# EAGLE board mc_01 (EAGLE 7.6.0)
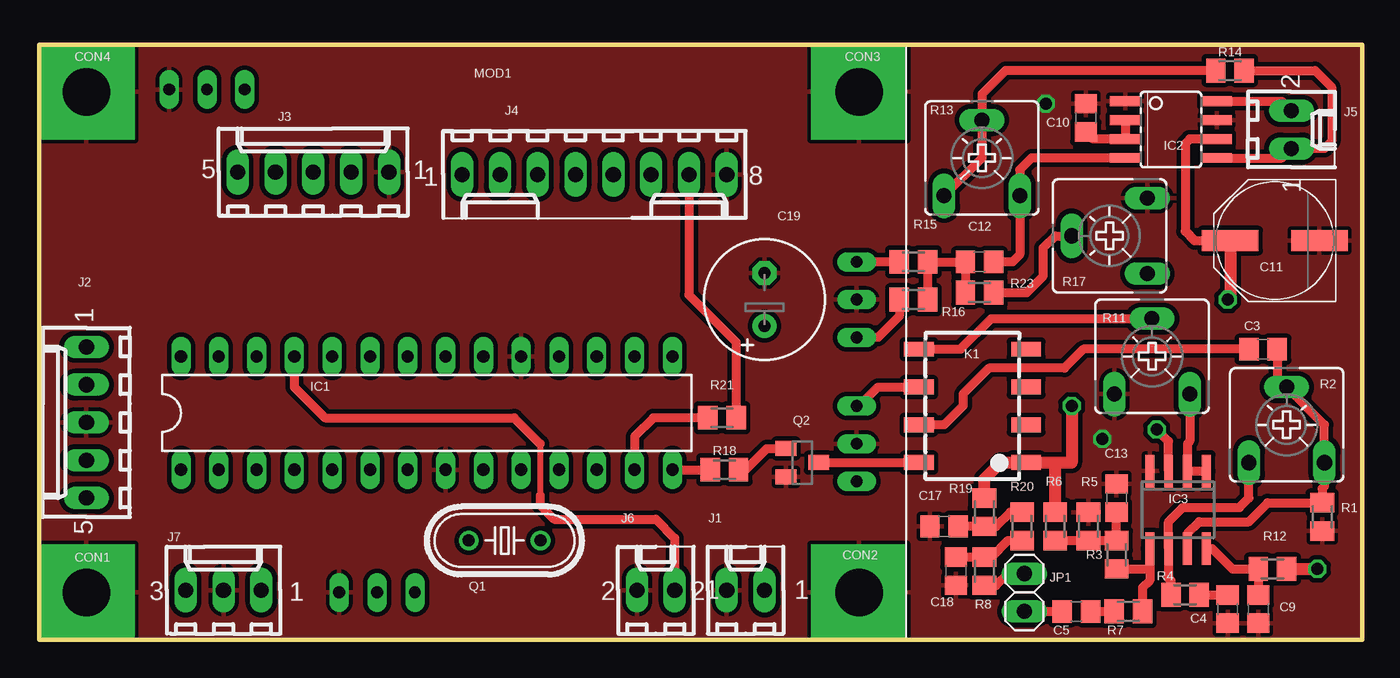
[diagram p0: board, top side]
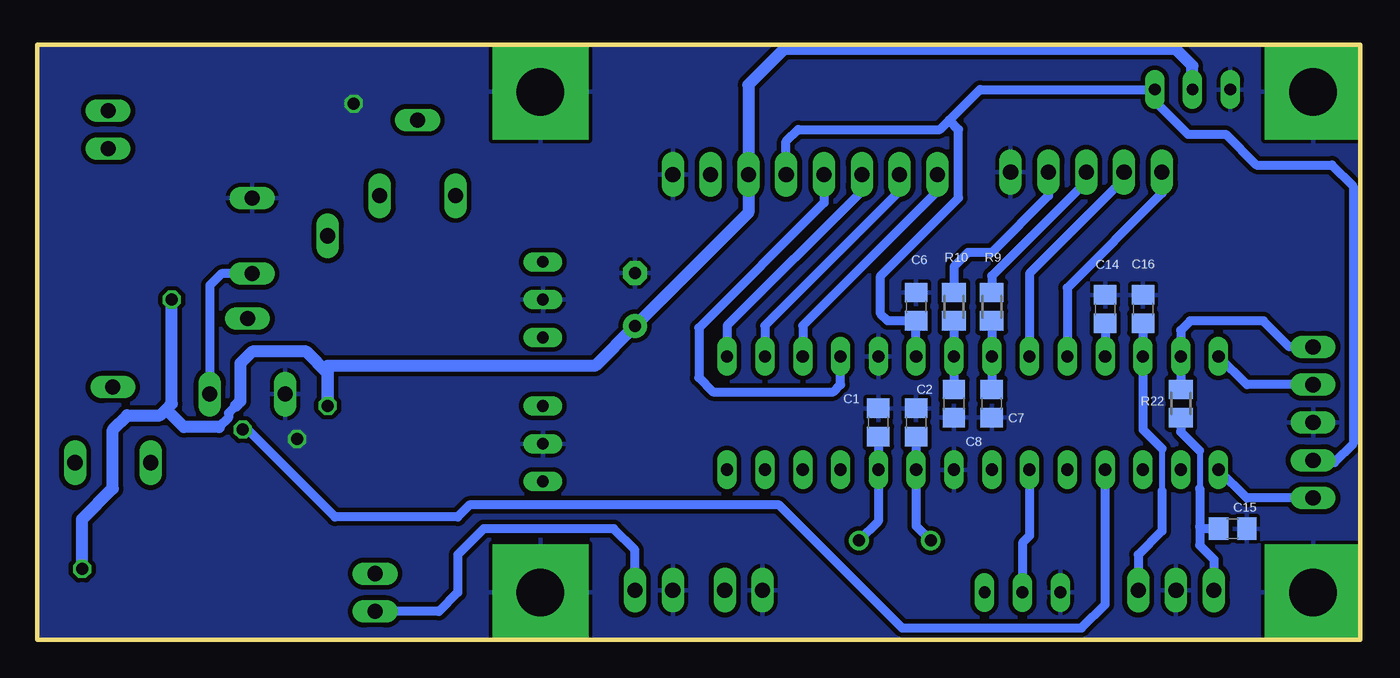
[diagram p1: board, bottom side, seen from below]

Size 88.9 x 40.01 mm. Coordinates in mm from the lower left corner, seen from the top.
Outline: 0,0 88.9,0 88.9,40.01 0,40.01 0,0
Copper layers (1*16): Top 0.035mm / dielectric 1.5mm / Bottom 0.035mm
Design rules "default *": minimum track width 10mil, minimum drill 24mil, track to track 8mil, track to pad 8mil, pad to pad 8mil, via to via 8mil, smd to smd 8mil, copper to edge 0mil, drill to drill 8mil, minimum pad ring 10mil, minimum via ring 8mil, stop-mask expansion 4mil, vias tented up to drill 0mil, thermal gap 10mil

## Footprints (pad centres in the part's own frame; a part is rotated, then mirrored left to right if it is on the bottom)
C0805 = smd 1.3 x 1.5: 1 -0.95,0; 2 0.95,0
PANASONIC_E = smd 3.8 x 1.4: + 3,0; - -3,0
E3,5-8 = drill 0.813 pad 1.6: + -1.778,0 | drill 0.813 pad 1.6 octagon: - 1.778,0
HOLE3 = drill 3.2 pad 6.452 square: 1 0,0
DIL28-3 = drill 0.813 long: 1 -16.51,-3.81; 2 -13.97,-3.81; 3 -11.43,-3.81; 4 -8.89,-3.81; 5 -6.35,-3.81; 6 -3.81,-3.81; 7 -1.27,-3.81; 8 1.27,-3.81; 9 3.81,-3.81; 10 6.35,-3.81; 11 8.89,-3.81; 12 11.43,-3.81; 13 13.97,-3.81; 14 16.51,-3.81; 15 16.51,3.81; 16 13.97,3.81; 17 11.43,3.81; 18 8.89,3.81; 19 6.35,3.81; 20 3.81,3.81; 21 1.27,3.81; 22 -1.27,3.81; 23 -3.81,3.81; 24 -6.35,3.81; 25 -8.89,3.81; 26 -11.43,3.81; 27 -13.97,3.81; 28 -16.51,3.81
SOIC08 = smd 0.66 x 2.032: 1 -1.905,-3.073; 2 -0.635,-3.073; 3 0.635,-3.073; 4 1.905,-3.073; 5 1.905,3.073; 6 0.635,3.073; 7 -0.635,3.073; 8 -1.905,3.073
SO08 = smd 0.6 x 2.2: 1 -1.905,-2.6; 2 -0.635,-2.6; 3 0.635,-2.6; 4 1.905,-2.6; 5 1.905,2.6; 6 0.635,2.6; 7 -0.635,2.6; 8 -1.905,2.6
6410-02 = drill 1.016 long: 1 1.27,0; 2 -1.27,0
6410-05 = drill 1.016 long: 1 5.08,0; 2 2.54,0; 3 0,0; 4 -2.54,0; 5 -5.08,0
6410-08 = drill 1.016 long: 1 8.89,0; 2 6.35,0; 3 3.81,0; 4 1.27,0; 5 -1.27,0; 6 -3.81,0; 7 -6.35,0; 8 -8.89,0
6410-03 = drill 1.016 long: 1 2.54,0; 2 0,0; 3 -2.54,0
1X02 = drill 1.016 long: 1 -1.27,0; 2 1.27,0
G6K-2F = smd 1 x 2: 1 -3.81,-3.6; 2 -1.27,-3.6; 3 1.27,-3.6; 4 3.81,-3.6; 5 3.81,3.6; 6 1.27,3.6; 7 -1.27,3.6; 8 -3.81,3.6
USB_QO100 = drill 0.8 long: 1 8.731,36.989; 2 11.271,36.989; 3 20.161,3.175; 4 22.701,3.175; 5 25.241,3.175; 6 54.928,25.4; 7 54.928,22.86; 8 54.928,20.32; 9 54.928,15.716; 10 54.928,13.176; 11 54.928,10.636; 12 13.811,36.989
HC49U-V = drill 0.813: 1 -2.413,0; 2 2.413,0
SOT23 = smd 1 x 1.4: 1 -0.95,-1.1; 2 0.95,-1.1; 3 0,1.1
M0805 = smd 1.3 x 1.6: 1 -0.95,0; 2 0.95,0
CA6V = drill 1.016 long: A -2.54,-2.54; E 2.54,-2.54; S 0,2.54

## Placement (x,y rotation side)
C1  27p  [C0805]  32.38,14.61 270 bottom
C2  27p  [C0805]  29.84,14.61 270 bottom
C3  1u  [C0805]  82.23,19.53 0 top
C4  10u  [C0805]  79.85,2.06 270 top
C5  1u  [C0805]  69.69,1.91 180 top
C6  100n  [C0805]  29.84,22.38 90 bottom
C7  100n  [C0805]  24.77,15.88 90 bottom
C8  100n  [C0805]  27.3,15.88 90 bottom
C9  10u  [C0805]  81.92,2.06 270 top
C10  1u  [C0805]  70.33,35.08 90 top
C11  47u  [PANASONIC_E]  83.03,26.83 180 top
C12  100n  [C0805]  63.18,25.4 180 top
C13  10u  [C0805]  72.39,9.53 270 top
C14  1n  [C0805]  17.14,22.23 270 bottom
C15  1n  [C0805]  8.57,7.46 0 bottom
C16  1n  [C0805]  14.61,22.23 270 bottom
C17  10u  [C0805]  60.8,7.62 0 top
C18  10u  [C0805]  61.59,4.6 90 top
C19  470u  [E3,5-8]  48.74,22.86 90 top
CON1  [HOLE3]  3.17,3.17 0 top
CON2  [HOLE3]  55.09,3.17 0 top
CON3  [HOLE3]  55.09,36.83 0 top
CON4  [HOLE3]  3.17,36.83 0 top
IC1  PIC18F26K22  [DIL28-3]  26.04,15.24 0 top
IC2  TPA4861  [SOIC08]  76.04,34.29 270 top
IC3  AD823  [SO08]  76.52,8.73 180 top
J1  Mike  [6410-02]  47.47,3.33 0 top
J2  Programmer  [6410-05]  3.17,14.61 90 top
J3  Drehgeber  [6410-05]  18.41,31.43 0 top
J4  LCD  [6410-08]  37.31,31.27 180 top
J5  LP  [6410-02]  84.14,34.29 270 top
J6  PTT  [6410-02]  41.43,3.33 0 top
J7  Keyer  [6410-03]  12.38,3.33 0 top
JP1  Speisung  [1X02]  66.2,3.17 270 top
K1  G6K-2F  [G6K-2F]  62.71,15.72 90 top
MOD1  USB-Modul  [USB_QO100]  0,0 0 top
Q1  16 MHz  [HC49U-V]  31.27,6.67 180 top
Q2  BSS123  [SOT23]  51.28,11.91 270 top
R1  10k  [M0805]  86.2,8.26 270 top
R2  22k  [CA6V]  83.82,14.45 0 top
R3  4,7k  [M0805]  72.39,5.71 90 top
R4  220  [M0805]  76.99,3.02 180 top
R5  4,7k  [M0805]  70.48,7.62 270 top
R6  4,7k  [M0805]  68.26,7.62 90 top
R7  1k  [M0805]  73.18,1.91 0 top
R8  2,2k  [M0805]  63.5,4.6 270 top
R9  100  [M0805]  24.77,22.38 90 bottom
R10  100  [M0805]  27.3,22.38 90 bottom
R11  50k  [CA6V]  74.77,19.05 0 top
R12  47  [M0805]  82.87,4.76 0 top
R13  100k  [CA6V]  63.34,32.38 0 top
R14  27k  [M0805]  80.01,38.26 0 top
R15  10k  [M0805]  58.74,25.4 0 top
R16  10k  [M0805]  58.74,22.86 0 top
R17  220k  [CA6V]  71.91,27.15 90 top
R18  4,7k  [M0805]  46.04,11.43 180 top
R19  1k  [M0805]  63.5,8.57 270 top
R20  1k  [M0805]  66.04,7.62 270 top
R21  180  [M0805]  45.88,14.92 0 top
R22  470  [M0805]  12.06,15.88 270 bottom
R23  10k  [M0805]  63.18,23.34 180 top

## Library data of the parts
C1-C19 R1 R3-R10 R12 R14-R16 R18-R23 = rcl
CON1-CON4 IC2 MOD1 = lindenau
IC1 = microchip; MF: MICROCHIP; MPN: PIC18F2550-I/SP; OC_FARNELL: 1523822; OC_NEWARK: 80K6054
IC3 = linear
J1-J7 = con-molex; OC_FARNELL: unknown; OC_NEWARK: unknown
JP1 = pinhead
K1 = relay; MF: OMRON COMPONENTS USA; MPN: G6K-2F DC24; OC_FARNELL: 1690427; OC_NEWARK: 36K7467
Q1 = crystal; OC_FARNELL: 1666969; OC_NEWARK: unknown
Q2 = transistor-small-signal
R2 R11 R13 R17 = pot

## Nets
5V: C11.+ C19.+ IC2.6 J4.6 K1.1 MOD1.2 R6.2 R12.2 R19.1
GND: C1.1 C2.1 C4.2 C6.2 C7.1 C8.1 C9.2 C10.2 C11.- C13.1 C14.1 C15.2 C16.1 C17.1 C18.1 C19.- CON1.1 CON2.1 CON3.1 CON4.1 IC1.8 IC1.19 IC2.1 IC2.7 IC3.4 J1.2 J2.3 J3.1 J4.8 J6.2 J7.2 MOD1.1 MOD1.3 MOD1.7 MOD1.10 Q2.2 R1.2 R5.1 R11.A R17.E
MCLR: IC1.1 J2.5
MIKE: C5.2 J1.1 JP1.2
N$1: J3.3 R9.2
N$2: IC3.1 IC3.2 R11.E R17.A
N$3: K1.6 MOD1.9
N$4: J3.2 R10.2
N$5: C10.1 IC2.2 IC2.3
N$6: R13.A R13.S R14.1
N$7: IC2.5 J5.1 R14.2
N$8: C9.1 IC3.8 R12.1
N$9: K1.5 R11.S
N$10: C2.2 IC1.9 Q1.2
N$11: C12.1 IC2.4 R13.E
N$12: C1.2 IC1.10 Q1.1
N$13: MOD1.6 R15.1
N$14: MOD1.8 R16.1
N$15: C12.2 R15.2 R16.2 R23.2
N$16: IC2.8 J5.2
N$17: K1.8 Q2.3
N$18: Q2.1 R18.1
N$19: C3.2 IC3.7 R1.1 R2.E R2.S
N$20: C18.2 R8.1 R20.2
N$21: C17.2 R19.2 R20.1
N$22: JP1.1 R8.2
N$23: J4.7 R21.2
N$24: R17.S R23.1
N$30: C5.1 R7.1
N$62: IC3.6 R2.A R4.2
N$63: C4.1 R4.1
N$64: C13.2 R3.2 R5.2 R6.1
N$65: IC3.5 R3.1 R7.2
N$76: C3.1 K1.7
RA0: IC1.2
RA1: IC1.3
RA2: IC1.4 IC3.3
RA3: IC1.5
RA4: IC1.6 MOD1.4
RA5: IC1.7
RB0: C8.2 IC1.21 R10.1
RB1: C7.2 IC1.22 R9.1
RB2: IC1.23 J3.4
RB3: IC1.24 J3.5
RB4: C14.2 IC1.25 J6.1
RB5: C16.2 IC1.26 J7.1
RB6: IC1.27 J2.1 R22.1
RB6_1: C15.1 J7.3 R22.2
RB7: IC1.28 J2.2
RC0: IC1.11
RC1: IC1.12
RC2: IC1.13 R21.1
RC3: IC1.14 R18.2
RC4: IC1.15 J4.3
RC5: IC1.16 J4.2
RC6: IC1.17 J4.1
RC7: IC1.18 J4.4
VDD: C6.1 IC1.20 J2.4 J4.5 MOD1.12

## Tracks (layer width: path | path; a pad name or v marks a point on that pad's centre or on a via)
5V  (via drill 0.8)
  Top 0.61: 66.2,11.8 K1.1 | IC2.6 77.31,33.66 76.99,33.34 76.99,27.46 77.63,26.83 C11.+
  Top 0.813: 68.1,11.91 K1.1 64.61,11.91 63.5,10.79 R19.1 | 68.1,11.91 69.37,11.91 v69.37,15.72 | R12.2 v85.88,4.76 | C11.+ 80.03,23.04 v79.85,22.86 | R6.2 68.26,11.75 68.1,11.91
  Bottom 0.61: 75.56,15.72 76.04,15.24 76.04,14.92 76.68,14.29
  Bottom 0.813: MOD1.2 11.27,38.58 12.38,39.69 38.73,39.69 41.12,37.31 J4.6 41.12,28.7 C19.+ 48.77,21.08 51.44,18.41 69.37,18.41 v69.37,15.72 69.37,17.94 70.8,19.37 74.45,19.37 75.25,18.57 75.25,16.03 75.56,15.72 | v85.88,4.76 85.88,8.1 83.82,10.16 83.82,14.13 82.87,15.08 80.64,15.08 80.25,15.48 | 80.25,15.48 79.85,15.88 v79.85,22.86 | 76.68,14.29 79.06,14.29 80.25,15.48
GND  (via drill 0.8)
  other vias: 71.44,13.49 67.63,36.04
  pour Bottom (isolate 0.305): 0,0 0,40.01 88.9,40.01 88.9,0
  pour Top (isolate 0.305): 0,0 0,40.01 88.9,40.01 88.9,0
MCLR
  Bottom 0.61: J2.5 7.62,9.53 IC1.1
MIKE
  Top 0.61: JP1.2 C5.2
  Bottom 0.61: J1.1 48.74,6.03 50.16,7.46 58.9,7.46 60.64,5.71 60.64,3.17 61.91,1.91 JP1.2
N$1
  Bottom 0.61: J3.3 18.41,30.8 24.77,24.45 R9.2
N$2
  Top 0.61: IC3.1 IC3.2 77.15,13.18 77.31,13.34 R11.E
  Bottom 0.61: R17.A 76.52,24.61 77.31,23.81 R11.E
N$3
  Top 0.61: MOD1.9 55.09,15.72 56.36,16.99 K1.6
N$4
  Bottom 0.61: J3.2 20.95,29.84 24.77,26.04 26.35,26.04 27.3,25.08 R10.2
N$5
  Top 0.61: C10.1 70.81,33.66 IC2.3 IC2.2
N$6
  Top 0.61: R13.A 63.34,32.38 R13.S 63.34,36.67 64.93,38.26 R14.1
N$7
  Top 0.61: IC2.5 83.5,32.38 J5.1 86.36,33.02 86.84,33.5 86.84,37.15 85.72,38.26 R14.2
N$8
  Top 0.61: 81.92,2.86 C9.1 R12.1 80.17,4.76 78.8,6.13 IC3.8
N$9
  Top 0.61: K1.5 61.91,19.53 63.98,21.59 R11.S 74.93,21.75
N$10
  Bottom 0.61: Q1.2 29.84,7.65 IC1.9 C2.2
N$11
  Top 0.61: C12.1 65.41,25.4 65.88,25.88 R13.E 65.88,31.59 66.67,32.38 IC2.4
N$12
  Bottom 0.61: Q1.1 32.38,7.97 IC1.10 C1.2
N$13
  Top 0.61: R15.1 MOD1.6
N$14
  Top 0.61: R16.1 57.79,21.75 56.36,20.32 MOD1.8
N$15
  Top 0.61: R16.2 R15.2 C12.2 R23.2
N$16
  Top 0.61: IC2.8 83.5,36.2 J5.2
N$17
  Top 0.61: Q2.3 K1.8
N$18
  Top 0.61: R18.1 47.47,11.43 48.9,12.86 Q2.1
N$19
  Top 0.61: IC3.7 77.15,7.14 77.95,7.94 81.28,7.94 82.55,9.21 R1.1 86.2,10.16 86.36,10.32 R2.E 86.36,14.45 R2.S 83.18,17.62 C3.2
N$20
  Top 0.61: C18.2 R8.1 63.97,5.55 65.09,6.67 R20.2
N$21
  Top 0.61: R20.1 65.24,8.57 64.29,7.62 R19.2 C17.2
N$22
  Top 0.61: R8.2 64.3,3.65 65.09,4.45 JP1.1
N$23
  Top 0.61: J4.7 43.66,23.18 46.83,20 R21.2
N$24
  Top 0.61: R23.1 66.36,23.34 67.47,24.45 67.47,26.35 68.26,27.15 R17.S
N$30
  Top 0.61: C5.1 R7.1
N$62
  Top 0.61: R2.A 81.28,9.53 80.64,8.89 76.83,8.89 75.88,7.94 IC3.6 75.88,4.13 76.04,3.97 R4.2
N$63
  Top 0.61: R4.1 C4.1
N$64
  Top 0.61: R6.1 R5.2 R3.2 C13.2
N$65
  Top 0.61: IC3.5 74.61,4.6 | 74.61,4.6 74.61,3.97 74.14,3.49 R7.2 | R3.1 74.45,4.76 74.61,4.6
N$76
  Top 0.61: C3.1 70.17,19.53 68.9,18.26 63.82,18.26 62.07,16.51 62.07,15.72 60.8,14.45 K1.7
RA2  (via drill 0.8)
  Top 0.61: IC3.3 75.88,13.34 v75.09,14.13
  Bottom 0.61: v75.09,14.13 74.77,14.13 68.9,8.26 60.64,8.26 59.85,9.05 39.05,9.05 30.8,0.79 18.73,0.79 17.14,2.38 IC1.4
RA4
  Bottom 0.61: IC1.6 22.23,6.99 22.7,6.51 MOD1.4
RB0
  Bottom 0.61: R10.1 IC1.21 C8.2
RB1
  Bottom 0.61: R9.1 IC1.22 C7.2
RB2
  Bottom 0.61: J3.4 15.88,30.96 22.23,24.61 IC1.23
RB3
  Bottom 0.61: J3.5 13.34,30 19.68,23.65 IC1.24
RB4
  Top 0.406: 33.66,13.18 33.66,9.68
  Top 0.61: IC1.25 17.14,16.99 19.21,14.92 31.91,14.92 33.66,13.18 | 33.66,9.68 33.66,9.05 34.61,8.1 41.43,8.1 42.7,6.83 J6.1
  Bottom 0.61: C14.2 IC1.25
RB5
  Bottom 0.406: 13.34,12.86 13.34,10
  Bottom 0.61: C16.2 IC1.26 14.61,14.13 13.34,12.86 | 13.34,10 13.34,7.3 14.92,5.71 J7.1
RB6
  Bottom 0.61: J2.1 4.76,19.68 6.51,21.43 11.43,21.43 12.06,20.8 IC1.27 R22.1
RB6_1
  Bottom 0.406: 10.79,12.7 10.79,10.16
  Bottom 0.61: R22.2 12.06,13.97 10.79,12.7 | 10.79,10.16 10.79,7.62 | 10.79,7.62 10.79,6.35 9.84,5.4 J7.3 | C15.1 10.64,7.46 10.79,7.62
RB7
  Bottom 0.61: J2.2 7.62,17.14 IC1.28
RC2
  Top 0.61: R21.1 41.27,14.92 40.01,13.65 IC1.13
RC3
  Top 0.61: IC1.14 R18.2
RC4
  Bottom 0.61: J4.3 33.5,30.16 42.55,21.11 IC1.15
RC5
  Bottom 0.61: J4.2 30.96,30.16 40.01,21.11 IC1.16
RC6
  Bottom 0.61: J4.1 28.42,30.16 37.47,21.11 IC1.17
RC7
  Bottom 0.61: J4.4 36.04,29.37 44.45,20.95 44.45,17.62 43.5,16.67 35.4,16.67 34.92,17.14 IC1.18
VDD
  Bottom 0.61: J4.5 38.58,33.5 37.78,34.29 28.26,34.29 27.62,34.92 | 27.62,34.92 25.56,36.99 MOD1.12 13.81,36.2 11.59,33.97 9.05,33.97 6.99,31.91 1.91,31.91 0.48,30.48 0.48,13.18 1.75,11.91 3.02,11.91 J2.4 | IC1.20 C6.1 31.75,21.43 32.23,21.91 32.23,24.45 26.99,29.69 26.99,34.29 27.62,34.92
